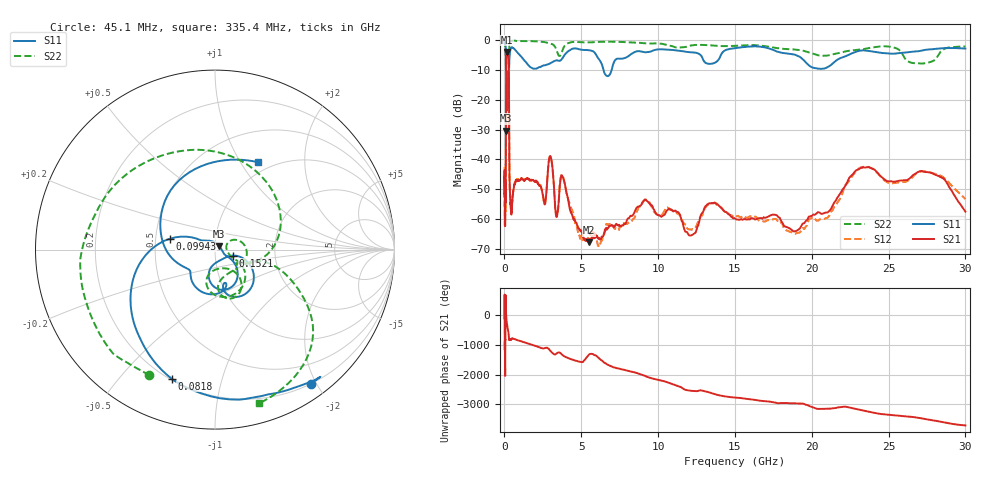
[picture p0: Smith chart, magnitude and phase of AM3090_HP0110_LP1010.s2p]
! Date/Time: Thu, Feb 28, 2019 2:00 PM
! Network Analyzer: Agilent Technologies E8364B Rev: A.07.50.67
! Sweep from 0.010 to 30.000 GHz, 1601 Points, Sweep Type: LOG
! Power Supply: 5.022 V, 0.002 A
# Hz S DB R 50
!freq MagS11 AngS11 MagS21 AngS21 MagS12 AngS12 MagS22 AngS22
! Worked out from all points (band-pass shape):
!   1601 points, 10 MHz to 30 GHz, reference 50 ohm
!   highest |S21| = -3.98 dB at 159.1 MHz (marker M1); lowest = -67.8 dB at 5.501 GHz (marker M2)
!   |S21| within 3 dB of the highest: 111.3 MHz to 271.5 MHz (160.2 MHz wide, 83.7 % of centre)
!   lowest |S11| = -30.4 dB at 107.7 MHz (marker M3), VSWR 1.06, Z = 52.3 + j2.09 ohm
!   |S11| at or under -10 dB: 98.35 MHz to 297.7 MHz (199.3 MHz wide, 101 % of centre); 6.447 GHz to 6.977 GHz (530.3 MHz wide, 7.9 % of centre)
!   |S22| runs from -23.9 to -0.2 dB; largest |S21 - S12| = 0.012
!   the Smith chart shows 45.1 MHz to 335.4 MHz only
!   S11 on the Smith chart (normalised r, x): 45.1 MHz: 0.20, -1.93; 81.8 MHz: 0.21, -0.70; 99.43 MHz: 0.60, +0.08; 152.1 MHz: 1.22, -0.08; 335.4 MHz: 0.87, +1.20
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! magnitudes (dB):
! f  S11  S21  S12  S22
! 10 MHz  -0.3  -45.7  -45.1  -0.6
! 38.04 MHz  -0.5  -58.6  -59.8  -1.5
! 45.1 MHz  -0.7  -58.3  -55.4  -2.1
! 81.8 MHz  -2.4  -52.1  -51.3  -4.7
! 99.43 MHz  -11.8  -16.9  -16.9  -11.2
! 107.7 MHz  -30.4  -8.3  -8.3  -23.3
! 123.3 MHz  -12.8  -5.3  -5.3  -15.9
! 144.7 MHz  -23.6  -4.2  -4.2  -17.0
! 152.1 MHz  -19.6  -4.0  -4.0  -16.7
! 159.1 MHz  -14.4  -4.0  -4.0  -14.9
! 274.6 MHz  -14.5  -7.5  -7.4  -16.2
! 335.4 MHz  -5.3  -47.7  -48.0  -1.0
! 550.5 MHz  -2.7  -51.9  -52.0  -0.3
! 2.084 GHz  -9.6  -47.5  -47.3  -0.5
! 3.002 GHz  -7.7  -39.1  -39.2  -1.2
! 3.385 GHz  -6.8  -59.2  -59.3  -3.4
! 3.798 GHz  -5.9  -45.9  -45.7  -3.2
! 5.501 GHz  -3.4  -67.8  -65.4  -0.8
! 7.926 GHz  -5.8  -61.1  -61.6  -0.7
! 18.93 GHz  -5.0  -64.1  -64.9  -3.2
! 23.48 GHz  -3.5  -42.8  -42.5  -2.9
! 30 GHz  -2.9  -57.5  -53.3  -2.2
